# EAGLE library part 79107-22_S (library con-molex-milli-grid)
RECEPTACAL
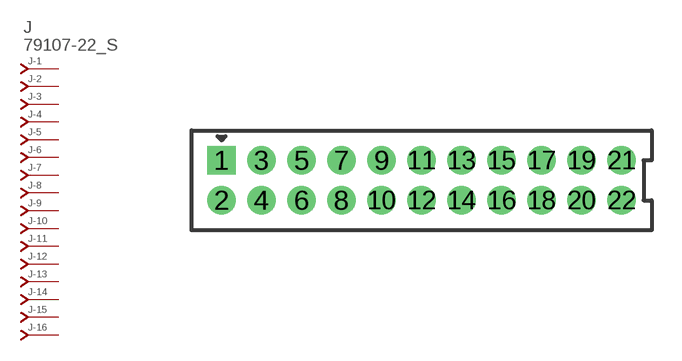
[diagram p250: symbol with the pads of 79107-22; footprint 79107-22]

Designator prefix J; gates -1=J-NV -2=J-N -3=J-N -4=J-N -5=J-N -6=J-N -7=J-N -8=J-N -9=J-N -10=J-N -11=J-N -12=J-N -13=J-N -14=J-N -15=J-N -16=J-N -17=J-N -18=J-N -19=J-N -20=J-N -21=J-N -22=J-N

## 79107-22_S  [79107-22]
1  -1:J  pas
2  -2:J  pas
3  -3:J  pas
4  -4:J  pas
5  -5:J  pas
6  -6:J  pas
7  -7:J  pas
8  -8:J  pas
9  -9:J  pas
10  -10:J  pas
11  -11:J  pas
12  -12:J  pas
13  -13:J  pas
14  -14:J  pas
15  -15:J  pas
16  -16:J  pas
17  -17:J  pas
18  -18:J  pas
19  -19:J  pas
20  -20:J  pas
21  -21:J  pas
22  -22:J  pas

## Footprint 79107-22 (pad centres in mm)
RECEPTACAL Dual Row, Vertical, Through-Hole
drill 0.914 square: 1 -10,1
drill 0.914: 2 -10,-1; 3 -8,1; 4 -8,-1; 5 -6,1; 6 -6,-1; 7 -4,1; 8 -4,-1; 9 -2,1; 10 -2,-1; 11 0,1; 12 0,-1; 13 2,1; 14 2,-1; 15 4,1; 16 4,-1; 17 6,1; 18 6,-1; 19 8,1; 20 8,-1; 21 10,1; 22 10,-1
